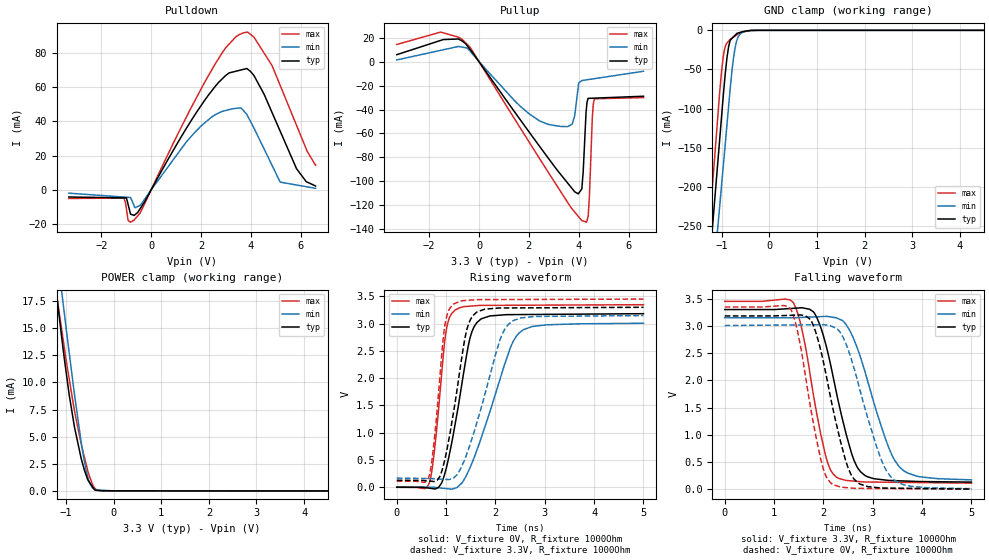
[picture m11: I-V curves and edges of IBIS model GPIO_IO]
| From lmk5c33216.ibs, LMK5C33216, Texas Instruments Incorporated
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[Model]   GPIO_IO
Model_type   I/O
Polarity   Non-Inverting
Enable   Active-Low
Vinl = 0.6
Vinh = 1.1
Vmeas = 1.65
Vref = 0
Cref = 2pF
Rref = 100000
|   typ   min   max
C_comp   1.6845E-12   1.6594E-12   1.6870E-12
| Where nom  PVT is Nominal Process, 3.3V,   27C
|   Fast PVT is Strong Process,  3.45V, -40C
|   Slow PVT is Weak Process,   3.15V, 125C
[Model spec]
|subparameter
Vinl   0.6   0.57   0.63
Vinh   1.1   1.05   1.15
[Voltage Range]   3.3   3.15   3.45
|Junction Temperature
[Temperature Range]   27   125   -40
[Pullup Reference]   3.3   3.15   3.45
[Pulldown Reference]   0   0   0
[Power Clamp Reference]   3.3   3.15   3.45
[GND Clamp Reference]   0   0   0
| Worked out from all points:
|   slope of the pulldown table from 0 to 0.495 V, typ, clamps not added: 38 ohm
|   slope of the pullup table from 0 to 0.495 V, typ, clamps not added: 33.8 ohm
|   GND clamp passes 1 mA (typ) near -0.50 V on its own axis
|   POWER clamp passes 1 mA (typ) near -0.54 V on its own axis
|   falling waveform, V_fixture 3.3V, R_fixture 1000Ohm: 20-80 % time 490ps typ, 620ps min, 403ps max; typ from 3.3 V to 0.131 V
|   rising waveform, V_fixture 0V, R_fixture 1000Ohm: 20-80 % time 366ps typ, 651ps min, 209ps max; typ from 0.003 V to 3.18 V
|   rising waveform, V_fixture 3.3V, R_fixture 1000Ohm: 20-80 % time 336ps typ, 562ps min, 198ps max; typ from 0.131 V to 3.3 V
|   falling waveform, V_fixture 0V, R_fixture 1000Ohm: 20-80 % time 470ps typ, 585ps min, 392ps max; typ from 3.18 V to 0.003 V
[Pulldown]
|   Voltage   I(typ)   I(min)   I(max)
-3.3V     -4.119mA   -1.898mA   -4.984mA
-1.087V   -4.62mA    -4.15mA    -4.728mA
-922.7mV  -8.493mA   -4.317mA   -17.77mA
-683.6mV  -14.85mA   -9.156mA   -17.57mA
-400.7mV  -10.06mA   -8.353mA   -12.29mA
2.427V    57.59mA    42.42mA    69.71mA
3.559V    69.68mA    47.76mA    90.57mA
3.872V    70.35mA    43.13mA    91.91mA
4.855V    45mA       14.24mA    72.37mA
5.18V     34.18mA    4.529mA    60.85mA
5.835V    12.37mA    2.873mA    37.64mA
6.6V      2.283mA    938.5uA    14.3mA
[GND Clamp]
|   Voltage   I(typ)   I(min)   I(max)
-3.3V     -1.815A    -1.777A    -1.852A
-1.266V   -302.4mA   -374.5mA   -252.1mA
-1.049V   -141.6mA   -226.7mA   -81.69mA
-973mV    -85.15mA   -174.8mA   -34.59mA
-929.8mV  -55.65mA   -145.5mA   -20.87mA
-859.1mV  -21.04mA   -97.37mA   -13.83mA
-825mV    -12.6mA    -74.12mA   -11.44mA
-757.1mV  -8.396mA   -35.86mA   -8.622mA
-683.5mV  -3.84mA    -12.55mA   -5.733mA
-579mV    -1.985mA   -2.982mA   -2.681mA
-229mV    -5.938uA   -15.66uA   -1.828uA
6.6V      0A         0A         0A
[Pullup]
|   Voltage   I(typ)   I(min)   I(max)
-3.3V     5.865mA    1.457mA    14.4mA
-683.6mV  17.4mA     12.22mA    18.76mA
2.75V     -79.84mA   -52.25mA   -91.51mA
3.735V    -106.1mA   -52.25mA   -123.2mA
3.983V    -110.5mA   -20.61mA   -129.3mA
4.125V    -106.3mA   -15.77mA   -132.9mA
4.317V    -37.41mA   -15.17mA   -134.3mA
4.382V    -30.68mA   -14.96mA   -128.9mA
4.434V    -30.64mA   -14.8mA    -110.5mA
4.546V    -30.55mA   -14.45mA   -46.8mA
4.63V     -30.48mA   -14.19mA   -31.04mA
6.6V      -28.89mA   -8.002mA   -30.04mA
[POWER Clamp]
|   Voltage   I(typ)   I(min)   I(max)
-3.3V     104.9mA    103mA      109.7mA
-1.21V    18.54mA    22.75mA    18.47mA
-1.137V   15.83mA    20.01mA    16.24mA
-1.054V   12.79mA    17.03mA    13.74mA
-934.9mV  8.882mA    12.76mA    10.37mA
-825mV    5.929mA    8.968mA    7.425mA
-684.4mV  3.026mA    4.552mA    4.375mA
-579.3mV  1.473mA    1.92mA     2.477mA
-492.1mV  691.2uA    605.6uA    1.17mA
-400.7mV  110.7uA    119.9uA    263uA
-259.3mV  12.38uA    67.95uA    14.88uA
6.6V      0A         0A         0A
[Ramp]
R_load = 1000
|   typ   min   max
dV/dt_r   1.90713/3.64846e-10   1.79879/6.47269e-10   2.00652/2.08519e-10
dV/dt_f   1.9005/4.88765e-10   1.78518/6.20012e-10   2.00201/4.0135e-10
[Falling Waveform]
V_fixture = 3.3V
V_fixture_min = 3.15V
V_fixture_max = 3.45V
R_fixture = 1000Ohm
C_fixture = 0F
|   Time   V(typ)   V(min)   V(max)
0s        3.299V     3.147V     3.449V
1.39ns    3.322V     3.148V     3.427V
1.599ns   3.326V     3.156V     2.793V
1.869ns   3.148V     3.167V     1.37V
2.088ns   2.516V     3.172V     482mV
2.261ns   1.786V     3.147V     225.2mV
2.698ns   388mV      2.566V     142.9mV
3.234ns   171.2mV    987.5mV    129.7mV
3.515ns   155.6mV    438.2mV    127mV
5ns       131.3mV    172.1mV    112.6mV
[Rising Waveform]
V_fixture = 0V
V_fixture_min = 0V
V_fixture_max = 0V
R_fixture = 1000Ohm
C_fixture = 0F
|   Time   V(typ)   V(min)   V(max)
0s        2.531mV    7.863mV    1.27mV
663.7ps   -15.34mV   3.842mV    95.78mV
786.6ps   -26.18mV   -888.8uV   868.8mV
989.2ps   305.8mV    -21.2mV    2.803V
1.179ns   1.142V     -14.12mV   3.244V
1.45ns    2.594V     292.1mV    3.317V
1.571ns   2.949V     550.7mV    3.325V
2.304ns   3.164V     2.56V      3.335V
2.483ns   3.165V     2.829V     3.336V
5ns       3.181V     3.006V     3.345V
[Rising Waveform]
V_fixture = 3.3V
V_fixture_min = 3.15V
V_fixture_max = 3.45V
R_fixture = 1000Ohm
C_fixture = 0F
|   Time   V(typ)   V(min)   V(max)
0s        130.7mV    170.5mV    112.3mV
656ps     116.3mV    161.5mV    212mV
769ps     110.4mV    157.8mV    950.5mV
969ps     489.4mV    147mV      2.935V
1.154ns   1.396V     173mV      3.357V
1.377ns   2.712V     511.9mV    3.422V
1.497ns   3.081V     818.6mV    3.43V
2.053ns   3.284V     2.591V     3.44V
2.26ns    3.286V     2.983V     3.441V
5ns       3.298V     3.147V     3.449V
[Falling Waveform]
|Gnd
V_fixture = 0V
V_fixture_min = 0V
V_fixture_max = 0V
R_fixture = 1000Ohm
C_fixture = 0F
|   Time   V(typ)   V(min)   V(max)
0s        3.181V     3.006V     3.346V
1.341ns   3.193V     3.016V     3.301V
1.523ns   3.199V     3.017V     2.693V
1.772ns   3.059V     3.019V     1.339V
1.999ns   2.342V     3.021V     370.6mV
2.16ns    1.623V     2.995V     107.6mV
2.62ns    188mV      2.227V     18.08mV
3.087ns   30.57mV    759.2mV    14.05mV
3.357ns   20.56mV    239mV      12.29mV
5ns       3.151mV    10.52mV    1.534mV
